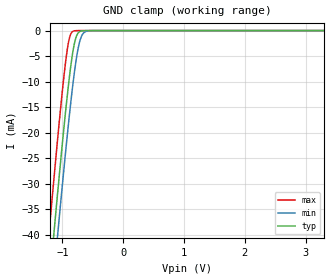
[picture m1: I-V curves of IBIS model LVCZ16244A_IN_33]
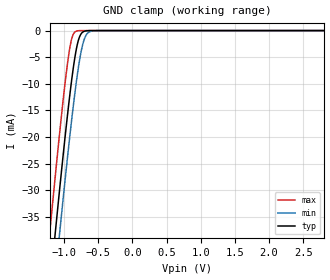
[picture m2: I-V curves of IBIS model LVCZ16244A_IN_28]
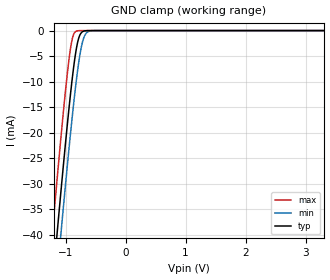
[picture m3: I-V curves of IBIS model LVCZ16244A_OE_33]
| TEXAS INSTRUMENTS INCORPORATED
| Standard Linear and Logic Group
| IBIS Model of SN74LVCZ16244A
| 16-BIT BUFFER/DRIVER WITH 3-STATE OUTPUTS
| This file contains package information for the following:
|  TSSOP 48-pin (DGG) package as [Component] LVCZ16244A_DGG
|  SSOP 48-pin (DL) package as [Component] LVCZ16244A_DL
| This device can be powered at the following Vccs:
|  3.3 volt Vcc
|  2.8 volt Vcc
| This file provides unique models under the [Model Selector] for each Vcc.
| For operation at a specific Vcc, select the appropriate model after each
| [Model Selector] keyword.
[IBIS Ver]   3.2
[Comment char]  |_char
[File Name]   sn74lvcz16244a.ibs
[File Rev]   1.1 | a_die
[Date]   August 28, 2002
[Source]   Data created from TI-SPICE simulations at TI-SLL.
[Notes]   The following is an IBIS list for the SN74LVCZ16244A.
   Please contact sllibis@ti.com with questions and
   comments concerning SLL IBIS models.
   - C_comp values are taken at a different test condition than
   the Ci in data sheet.
   - C_comp values are taken at a different test condition than
   the Co in data sheet.
[Disclaimer] Property of Texas Instruments Incorporated. Unauthorized
   reproduction and/or distribution is strictly prohibited.
   This product is protected under copyright law.
   Created 2002, (C) Copyright 2002, Texas Instruments
   Incorporated, All Rights Reserved
   UNLESS THERE IS A SIGNED, WRITTEN AGREEMENT TO THE
   CONTRARY, TEXAS INSTRUMENTS (TI) IS PROVIDING THE IBIS
   MODELS AND WITHOUT ANY WARRANTY, EXPRESSED OR
   IMPLIED. TI assumes no liability for:
   1) the accuracy of the IBIS models provided to your
   company;
   2) the proper functioning of these IBIS Models in your
   design or for any resulting applications; or
   3) infringement of patents, copyrights or intellectual
   property rights resulting from your use of these IBIS
   models.
   TI provides IBIS Models as a service to our customers.
   You and your company shall not distribute, sell or give
   these models to anyone else without prior written
   permission from TI.
   TI reserves the right to make changes to our products or
   to discontinue any semiconductor product or service
   without notice, and advises our customers to obtain the
   latest version of relevant information to verify, before
   placing orders, that the information being relied on is
   current.
   Please be aware that your receipt and use of the IBIS
   information provided shall serve as acceptance of these
   terms and conditions. If you do not accept these terms,
   you should return or destroy the IBIS models and any
   other accompanying information immediately.
| Component LVCZ16244A_DGG 48-pin TSSOP
[Component]   LVCZ16244A_DGG
[Manufacturer]  Texas Instruments, Inc.
[Package]
|   typ   min   max
R_pkg   6.200e-02   5.000e-02   7.800e-02
L_pkg   3.527e-09   3.128e-09   4.255e-09
C_pkg   5.300e-13   4.170e-13   6.850e-13
[Pin]   signal_name   model_name   R_pin   L_pin   C_pin
1   1NOE   LVCZ16244A_OE   5.000e-02   4.250e-09   6.710e-13
2   1Y1   LVCZ16244A_OUT   5.700e-02   3.956e-09   6.740e-13
3   1Y2   LVCZ16244A_OUT   7.100e-02   3.922e-09   6.190e-13
4   GND   GND   7.800e-02   3.841e-09   6.180e-13
5   1Y3   LVCZ16244A_OUT   5.600e-02   3.535e-09   5.550e-13
6   1Y4   LVCZ16244A_OUT   5.800e-02   3.464e-09   5.030e-13
7   VCC   POWER   6.000e-02   3.362e-09   4.980e-13
8   2Y1   LVCZ16244A_OUT   6.100e-02   3.293e-09   4.620e-13
9   2Y2   LVCZ16244A_OUT   6.300e-02   3.240e-09   4.550e-13
10   GND   GND   6.300e-02   3.175e-09   4.420e-13
11   2Y3   LVCZ16244A_OUT   6.400e-02   3.153e-09   4.290e-13
12   2Y4   LVCZ16244A_OUT   6.500e-02   3.128e-09   4.180e-13
13   3Y1   LVCZ16244A_OUT   6.500e-02   3.128e-09   4.180e-13
14   3Y2   LVCZ16244A_OUT   6.400e-02   3.154e-09   4.290e-13
15   GND   GND   6.300e-02   3.174e-09   4.420e-13
16   3Y3   LVCZ16244A_OUT   6.300e-02   3.241e-09   4.550e-13
17   3Y4   LVCZ16244A_OUT   6.100e-02   3.293e-09   4.620e-13
18   VCC   POWER   6.000e-02   3.362e-09   4.970e-13
19   4Y1   LVCZ16244A_OUT   5.800e-02   3.464e-09   5.030e-13
20   4Y2   LVCZ16244A_OUT   5.600e-02   3.537e-09   5.600e-13
21   GND   GND   7.700e-02   3.839e-09   6.260e-13
22   4Y3   LVCZ16244A_OUT   7.100e-02   3.917e-09   6.270e-13
23   4Y4   LVCZ16244A_OUT   5.800e-02   3.955e-09   6.850e-13
24   4NOE   LVCZ16244A_OE   5.200e-02   4.255e-09   6.790e-13
25   3NOE   LVCZ16244A_OE   5.100e-02   4.254e-09   6.760e-13
26   4A4   LVCZ16244A_IN   5.800e-02   3.957e-09   6.790e-13
27   4A3   LVCZ16244A_IN   7.100e-02   3.920e-09   6.210e-13
28   GND   GND   7.800e-02   3.843e-09   6.220e-13
29   4A2   LVCZ16244A_IN   5.600e-02   3.539e-09   5.600e-13
30   4A1   LVCZ16244A_IN   5.800e-02   3.466e-09   5.030e-13
31   VCC   POWER   6.000e-02   3.363e-09   4.970e-13
32   3A4   LVCZ16244A_IN   6.100e-02   3.294e-09   4.620e-13
33   3A3   LVCZ16244A_IN   6.300e-02   3.241e-09   4.540e-13
34   GND   GND   6.300e-02   3.175e-09   4.410e-13
35   3A2   LVCZ16244A_IN   6.400e-02   3.153e-09   4.290e-13
36   3A1   LVCZ16244A_IN   6.500e-02   3.129e-09   4.170e-13
37   2A4   LVCZ16244A_IN   6.500e-02   3.129e-09   4.170e-13
38   2A3   LVCZ16244A_IN   6.400e-02   3.152e-09   4.290e-13
39   GND   GND   6.400e-02   3.176e-09   4.410e-13
40   2A2   LVCZ16244A_IN   6.300e-02   3.241e-09   4.540e-13
41   2A1   LVCZ16244A_IN   6.100e-02   3.293e-09   4.620e-13
42   VCC   POWER   6.000e-02   3.363e-09   4.970e-13
43   1A4   LVCZ16244A_IN   5.800e-02   3.464e-09   5.030e-13
44   1A3   LVCZ16244A_IN   5.600e-02   3.534e-09   5.610e-13
45   GND   GND   7.800e-02   3.841e-09   6.260e-13
46   1A2   LVCZ16244A_IN   7.100e-02   3.920e-09   6.220e-13
47   1A1   LVCZ16244A_IN   5.700e-02   3.955e-09   6.770e-13
48   2NOE   LVCZ16244A_OE   5.100e-02   4.252e-09   6.720e-13
| Component LVCZ16244A_DL 48-pin SSOP
[Component]   LVCZ16244A_DL
[Manufacturer]   Texas Instruments, Inc.
[Package]
|   typ   min   max
R_pkg   4.800e-02   3.800e-02   5.300e-02
L_pkg   6.046e-09   5.084e-09   7.968e-09
C_pkg   8.130e-13   5.690e-13   1.157e-12
[Pin]   signal_name   model_name   R_pin   L_pin   C_pin
1   1NOE   LVCZ16244A_OE   4.600e-02   7.968e-09   1.017e-12
2   1Y1   LVCZ16244A_OUT   4.400e-02   7.299e-09   1.157e-12
3   1Y2   LVCZ16244A_OUT   4.300e-02   6.765e-09   1.058e-12
4   GND   GND   4.100e-02   6.269e-09   9.330e-13
5   1Y3   LVCZ16244A_OUT   3.800e-02   5.856e-09   8.290e-13
6   1Y4   LVCZ16244A_OUT   4.600e-02   5.802e-09   7.900e-13
7   VCC   POWER   5.000e-02   5.656e-09   7.380e-13
8   2Y1   LVCZ16244A_OUT   5.300e-02   5.500e-09   6.430e-13
9   2Y2   LVCZ16244A_OUT   5.200e-02   5.304e-09   6.060e-13
10   GND   GND   5.300e-02   5.189e-09   5.830e-13
11   2Y3   LVCZ16244A_OUT   5.100e-02   5.084e-09   5.690e-13
12   2Y4   LVCZ16244A_OUT   5.300e-02   5.862e-09   8.330e-13
13   3Y1   LVCZ16244A_OUT   5.300e-02   5.862e-09   8.330e-13
14   3Y2   LVCZ16244A_OUT   5.100e-02   5.084e-09   5.690e-13
15   GND   GND   5.300e-02   5.189e-09   5.830e-13
16   3Y3   LVCZ16244A_OUT   5.200e-02   5.304e-09   6.060e-13
17   3Y4   LVCZ16244A_OUT   5.300e-02   5.500e-09   6.430e-13
18   VCC   POWER   5.000e-02   5.656e-09   7.380e-13
19   4Y1   LVCZ16244A_OUT   4.600e-02   5.802e-09   7.900e-13
20   4Y2   LVCZ16244A_OUT   3.800e-02   5.856e-09   8.290e-13
21   GND   GND   4.100e-02   6.269e-09   9.330e-13
22   4Y3   LVCZ16244A_OUT   4.300e-02   6.765e-09   1.058e-12
23   4Y4   LVCZ16244A_OUT   4.400e-02   7.299e-09   1.157e-12
24   4NOE   LVCZ16244A_OE   4.600e-02   7.968e-09   1.017e-12
25   3NOE   LVCZ16244A_OE   4.600e-02   7.968e-09   1.017e-12
26   4A4   LVCZ16244A_IN   4.400e-02   7.299e-09   1.157e-12
27   4A3   LVCZ16244A_IN   4.300e-02   6.765e-09   1.058e-12
28   GND   GND   4.100e-02   6.269e-09   9.330e-13
29   4A2   LVCZ16244A_IN   3.800e-02   5.856e-09   8.290e-13
30   4A1   LVCZ16244A_IN   4.600e-02   5.802e-09   7.900e-13
31   VCC   POWER   5.000e-02   5.656e-09   7.380e-13
32   3A4   LVCZ16244A_IN   5.300e-02   5.500e-09   6.430e-13
33   3A3   LVCZ16244A_IN   5.200e-02   5.304e-09   6.060e-13
34   GND   GND   5.300e-02   5.189e-09   5.830e-13
35   3A2   LVCZ16244A_IN   5.100e-02   5.084e-09   5.690e-13
36   3A1   LVCZ16244A_IN   5.300e-02   5.862e-09   8.330e-13
37   2A4   LVCZ16244A_IN   5.300e-02   5.862e-09   8.330e-13
38   2A3   LVCZ16244A_IN   5.100e-02   5.084e-09   5.690e-13
39   GND   GND   5.300e-02   5.189e-09   5.830e-13
40   2A2   LVCZ16244A_IN   5.200e-02   5.304e-09   6.060e-13
41   2A1   LVCZ16244A_IN   5.300e-02   5.500e-09   6.430e-13
42   VCC   POWER   5.000e-02   5.656e-09   7.380e-13
43   1A4   LVCZ16244A_IN   4.600e-02   5.802e-09   7.900e-13
44   1A3   LVCZ16244A_IN   3.800e-02   5.856e-09   8.290e-13
45   GND   GND   4.100e-02   6.269e-09   9.330e-13
46   1A2   LVCZ16244A_IN   4.300e-02   6.765e-09   1.058e-12
47   1A1   LVCZ16244A_IN   4.400e-02   7.299e-09   1.157e-12
48   2NOE   LVCZ16244A_OE   4.600e-02   7.967e-09   1.017e-12
| Model LVCZ16244A_IN
[Model Selector]   LVCZ16244A_IN
LVCZ16244A_IN_33   3.3 volt Vcc
LVCZ16244A_IN_28   2.8 volt Vcc
| Model LVCZ16244A_OE
[Model Selector]   LVCZ16244A_OE
LVCZ16244A_OE_33   3.3 volt Vcc
LVCZ16244A_OE_28   2.8 volt Vcc
| Model LVCZ16244A_OUT
[Model Selector]   LVCZ16244A_OUT
LVCZ16244A_OUT_33   3.3 volt Vcc
LVCZ16244A_OUT_28   2.8 volt Vcc
| Models and submodels in the file (6): LVCZ16244A_IN_33 (Input), LVCZ16244A_IN_28 (Input), LVCZ16244A_OE_33 (Input), LVCZ16244A_OE_28 (Input), LVCZ16244A_OUT_33 (3-state), LVCZ16244A_OUT_28 (3-state)
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[Model]   LVCZ16244A_IN_33
Model_type  Input
Vinl=0.8
Vinh=2
| variable   typ   min   max
C_comp   3.32pF   2.61pF   4.29pF
[Temperature Range]   40   100   -40
| Ambient temperature   25   85   -40
[Voltage range]   3.3   3   3.6
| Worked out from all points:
|   GND clamp passes 1 mA (typ) near -0.77 V on its own axis
[GND Clamp]
| LVCZ16244A_IN_33
|   Voltage   I(typ)   I(min)   I(max)
-5V       -583.8mA   -590.8mA   -575.1mA
-1.215V   -49.6mA    -57.88mA   -38.96mA
-1.14V    -39.72mA   -48.01mA   -29.07mA
-1.08V    -31.98mA   -40.25mA   -21.38mA
-1.06V    -29.44mA   -37.69mA   -18.89mA
-925mV    -13.29mA   -21.11mA   -4.122mA
-875mV    -8.124mA   -15.45mA   -1.065mA
-820mV    -3.579mA   -9.774mA   -109.4uA
-770mV    -1.128mA   -5.445mA   -10.73uA
-715mV    -205.4uA   -2.128mA   -808.5nA
-590mV    -2.7uA     -81.86uA   -2.255nA
3.3V      6.304pA    9.258pA    5.93pA
[Model]   LVCZ16244A_IN_28
Model_type  Input
Vinl=0.8
Vinh=2
| variable   typ   min   max
C_comp   3.37pF   2.65pF   4.28pF
[Temperature Range]   40   100   -40
| Ambient temperature   25   85   -40
[Voltage range]   2.8   2.7   2.9
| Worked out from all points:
|   GND clamp passes 1 mA (typ) near -0.77 V on its own axis
[GND Clamp]
| LVCZ16244A_IN_28
|   Voltage   I(typ)   I(min)   I(max)
-5V       -583.8mA   -590.8mA   -575.1mA
-1.205V   -48.27mA   -56.56mA   -37.63mA
-1.13V    -38.42mA   -46.71mA   -27.77mA
-1.07V    -30.71mA   -38.96mA   -20.13mA
-1.05V    -28.19mA   -36.42mA   -17.65mA
-955mV    -16.68mA   -24.66mA   -6.874mA
-885mV    -9.098mA   -16.55mA   -1.486mA
-830mV    -4.281mA   -10.75mA   -171.6uA
-780mV    -1.472mA   -6.227mA   -17.15uA
-710mV    -173.7uA   -1.918mA   -639nA
-645mV    -18.49uA   -387.7uA   -29.98nA
2.8V      5.31pA     8.079pA    5.035pA
[Model]   LVCZ16244A_OE_33
Model_type  Input
Vinl=0.8
Vinh=2
| variable   typ   min   max
C_comp   3.79pF   2.92pF   4.89pF
[Temperature Range]   40   100   -40
| Ambient temperature   25   85   -40
[Voltage range]   3.3   3   3.6
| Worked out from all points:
|   GND clamp passes 1 mA (typ) near -0.77 V on its own axis
[GND Clamp]
| LVCZ16244A_OE_33
|   Voltage   I(typ)   I(min)   I(max)
-5V       -583.8mA   -590.8mA   -575.1mA
-1.215V   -49.6mA    -57.88mA   -38.96mA
-1.14V    -39.72mA   -48.01mA   -29.07mA
-1.08V    -31.98mA   -40.25mA   -21.38mA
-1.06V    -29.44mA   -37.69mA   -18.89mA
-925mV    -13.29mA   -21.11mA   -4.122mA
-875mV    -8.124mA   -15.45mA   -1.065mA
-820mV    -3.579mA   -9.774mA   -109.4uA
-770mV    -1.128mA   -5.445mA   -10.73uA
-715mV    -205.4uA   -2.128mA   -808.5nA
-590mV    -2.7uA     -81.86uA   -2.255nA
3.3V      6.304pA    9.258pA    5.93pA
